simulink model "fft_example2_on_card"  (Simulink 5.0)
settings: Solver=ode45  StartTime=0.0  StopTime=100000.0  RelTol=1e-3
undefined symbols (not defined in the file or in its folder): get
libraries: ADlibrary x2, dspsigattribs x2, dspsnks4 x2, simulink x1

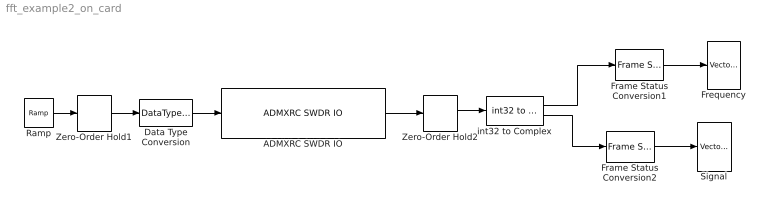
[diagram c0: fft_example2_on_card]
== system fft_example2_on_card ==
  ADMXRC SWDR IO : ADlibrary/Hardware in the Loop/ADMXRC SWDR IO  AncestorBlock=ADlibrary/ADMXRC Slave I//O  filename=e:\tmp5\fft_example2.bit  clock_freq=33  mclk_freq=25  input_width=1  output_width=64  index=0
  Data Type Conversion : DataTypeConversion  DataType=uint32
  Frame Status Conversion1 : dspsigattribs/Frame Status Conversion  growRefPort=off  outframe=Frame-based
  Frame Status Conversion2 : dspsigattribs/Frame Status Conversion  growRefPort=off  outframe=Frame-based
  Frequency : dspsnks4/Vector Scope  ScopeProperties=on  Domain=User-defined  HorizSpan=1  DisplayProperties=off  AxisGrid=on  Memory=off  FrameNumber=on  AxisLegend=off  AxisZoom=off  OpenScopeAtSimStart=on  OpenScopeImmediately=off  FigPos=get(0,'defaultfigureposition')  AxisProperties=off  XUnits=Hertz  XRange=[0...Fs/2]  InheritXIncr=on  XIncr=1  XLabel=Frequency  YUnits=dB  YLabel=Magnitude  LineProperties=off
  Ramp : simulink/Sources/Ramp  slope=0.01  start=0  X0=8
  Signal : dspsnks4/Vector Scope  ScopeProperties=on  Domain=User-defined  HorizSpan=1  DisplayProperties=off  AxisGrid=on  Memory=off  FrameNumber=on  AxisLegend=off  AxisZoom=off  OpenScopeAtSimStart=on  OpenScopeImmediately=off  FigPos=get(0,'defaultfigureposition')  AxisProperties=off  XUnits=Hertz  XRange=[0...Fs/2]  InheritXIncr=on  XIncr=1  XLabel=Frequency  YUnits=dB  YLabel=Magnitude  LineProperties=off
  Zero-Order Hold1 : ZeroOrderHold
  Zero-Order Hold2 : ZeroOrderHold  SampleTime=70
  int32 to Complex : ADlibrary/Miscellaneous/int32 to Complex
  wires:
  Ramp/1 -> Zero-Order Hold1/1
  Zero-Order Hold1/1 -> Data Type Conversion/1
  Data Type Conversion/1 -> ADMXRC SWDR IO/1
  ADMXRC SWDR IO/1 -> Zero-Order Hold2/1
  Zero-Order Hold2/1 -> int32 to Complex/1
  Frame Status Conversion1/1 -> Frequency/1
  Frame Status Conversion2/1 -> Signal/1
  int32 to Complex/1 -> Frame Status Conversion1/1
  int32 to Complex/2 -> Frame Status Conversion2/1
